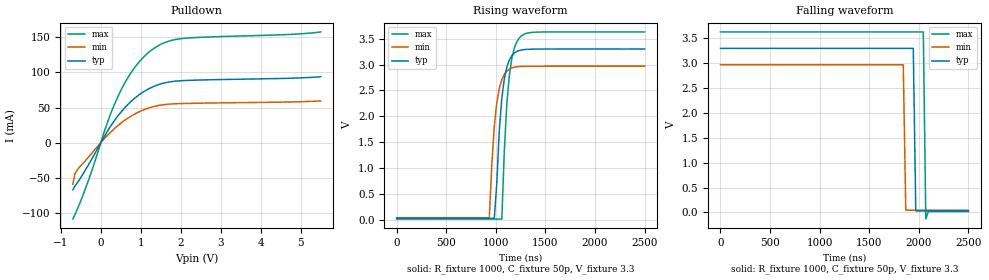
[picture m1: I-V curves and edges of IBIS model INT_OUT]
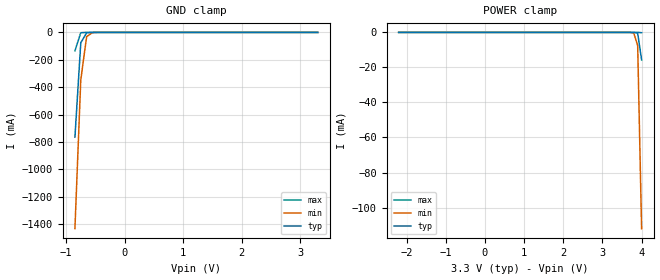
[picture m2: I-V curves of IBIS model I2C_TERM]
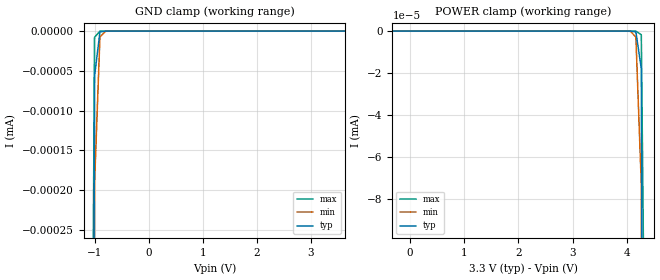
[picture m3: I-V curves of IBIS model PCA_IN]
|   NXP Semiconductors Inc.
|   Specialty Logic Products Group
|   IBIS model of PCA9545B
|   4-Channel I2C switch with
|   interrupt logic and reset
[IBIS Ver]   3.2
[Comment Char]   |_char
|  VDD Typ: 3.3V, Min: 2.97V, Max: 3.63V
[File name]   pca9545b_3_3v.ibs
[File Rev]   1.0
[Date]   Dec 05, 2007 1:30:50 PM
[Source]
Generated by Seshadri Venkataramanan with IbisToolKit at Tempe, AZ
[Notes]
[Disclaimer]
(C) Copyright 2007 NXP Semiconductors
All rights reserved
NXP Semiconductors (NXP) does not warrant that this model and any other
accompanying information (Model) accurately or fully represents the
operating characteristics and specifications of the semiconductor
products to which the Model relates.  Moreover, the Model is furnished
on an "as is" and with "all faults" basis, and without support or
warranty of any kind.  NXP disclaims all warranties, whether expressed
or implied or statutory, including without limitation all implied
warranties of non-infringement, merchantability and fitness for any
purpose, and those arising from a course of dealing or usage of trade.
NXP does not convey any license under its or any third party's patents,
copyrights or other intellectual property or proprietary rights.
You and your company assume any and all risks and liability arising out
of the application or use of the Model.
In no event shall NXP be liable for any direct, indirect, special,
consequential or incidental damages, however caused, whether in
warranty, contract or tort (including negligence), strict liability or
other legal theory, including, without limitation, for lost profits,
business interruption, or corruption or loss of data or information,
arising out of or in connection with the use of or the inability to use
the Model, even if NXP has been advised of the possibility of such
damages.
NXP provides the Model as a courtesy to our customers. You and your
company shall not distribute, convey, sell, or give the Model to anyone
else without receiving prior written permission from NXP.
NXP reserves the right to make changes without notice to the Model to
improve reliability, function, or design.
Please be aware that your receipt and subsequent use of the Model shall
serve as acceptance of these terms and conditions.  If you do not
accept these terms, return or destroy the Model immediately.
[Copyright]
2007
[Component]   PCA9545AD
Si_location Pin
Timing_location Pin
[Manufacturer]   NXP Semiconductors
[Package]
|   variable   typ   min   max
R_pkg   5.95E-02   5.36E-02   6.59E-02
L_pkg   4.21E-09   3.07E-09   5.91E-09
C_pkg   0.910E-12   0.758E-12   1.110E-12
|   SO20
[Pin] signal_name   model_name   R_pin   L_pin   C_pin
1   A0   PCA_IN   5.75E-02  5.91E-09  1.050E-12
2   A1   PCA_IN   6.25E-02  4.85E-09  1.040E-12
3   RESETB   PCA_IN   6.59E-02  3.92E-09  0.861E-12
4   INT0B   INT_IN   5.79E-02  3.32E-09  0.803E-12
5   SD0   I2C_TERM   5.36E-02  3.07E-09  0.758E-12
6   SC0   I2C_TERM   5.36E-02  3.07E-09  0.758E-12
7   INT1B   INT_IN   5.79E-02  3.32E-09  0.803E-12
8   SD1   I2C_TERM   6.59E-02  3.92E-09  0.861E-12
9   SC1   I2C_TERM   6.25E-02  4.85E-09  1.040E-12
10   Vss   GND   5.75E-02  5.91E-09  1.110E-12
11   INT2B   INT_IN   5.75E-02  5.91E-09  1.110E-12
12   SD2   I2C_TERM   6.25E-02  4.85E-09  1.040E-12
13   SC2   I2C_TERM   6.59E-02  3.92E-09  0.861E-12
14   INT3B   INT_IN   5.79E-02  3.32E-09  0.803E-12
15   SD3   I2C_TERM   5.36E-02  3.07E-09  0.758E-12
16   SC3   I2C_TERM   5.36E-02  3.07E-09  0.758E-12
17   INTB   INT_OUT   5.79E-02  3.32E-09  0.803E-12
18   SCL   I2C_TERM   6.59E-02  3.92E-09  0.861E-12
19   SDA   I2C_TERM   6.25E-02  4.85E-09  1.040E-12
20   Vdd   POWER   5.75E-02  5.91E-09  1.110E-12
[Component]   PCA9545APW
Si_location Pin
Timing_location Pin
[Manufacturer]   NXP Semiconductors
[Package]
|   variable   typ   min   max
R_pkg   7.24E-02   6.63E-02   8.34E-02
L_pkg   2.47E-09   2.09E-09   3.18E-09
C_pkg   0.341E-12   0.282E-12   0.420E-12
|   TSSOP20
[Pin] signal_name   model_name   R_pin   L_pin   C_pin
1   A0   PCA_IN   6.63E-02  3.18E-09  0.408E-12
2   A1   PCA_IN   6.67E-02  2.55E-09  0.398E-12
3   RESETB   PCA_IN   8.34E-02  2.35E-09  0.317E-12
4   INT0B   INT_IN   7.44E-02  2.16E-09  0.293E-12
5   SD0   I2C_TERM   7.10E-02  2.09E-09  0.282E-12
6   SC0   I2C_TERM   7.10E-02  2.09E-09  0.282E-12
7   INT1B   INT_IN   7.44E-02  2.16E-09  0.293E-12
8   SD1   I2C_TERM   8.34E-02  2.35E-09  0.317E-12
9   SC1   I2C_TERM   6.67E-02  2.55E-09  0.397E-12
10   Vss   GND   6.63E-02  3.18E-09  0.420E-12
11   INT2B   INT_IN   6.63E-02  3.17E-09  0.420E-12
12   SD2   I2C_TERM   6.67E-02  2.55E-09  0.397E-12
13   SC2   I2C_TERM   8.34E-02  2.35E-09  0.317E-12
14   INT3B   INT_IN   7.44E-02  2.16E-09  0.293E-12
15   SD3   I2C_TERM   7.10E-02  2.09E-09  0.282E-12
16   SC3   I2C_TERM   7.10E-02  2.09E-09  0.282E-12
17   INTB   INT_OUT   7.44E-02  2.16E-09  0.293E-12
18   SCL   I2C_TERM   8.34E-02  2.35E-09  0.317E-12
19   SDA   I2C_TERM   6.67E-02  2.55E-09  0.398E-12
20   Vdd   POWER   6.63E-02  3.17E-09  0.420E-12
[Component]   PCA9545ABS
Si_location Pin
Timing_location Pin
[Manufacturer]   NXP Semiconductors
[Package]
|   variable   typ   min   max
R_pkg   0.364   0.215   0.513
L_pkg   1.49E-09   1.04E-09   1.93E-09
C_pkg   0.149E-12   0.124E-12   0.173E-12
|   HVQFN20
[Package Model]   hvqfn20
[Pin] signal_name   model_name
1   RESETB   I2C_TERM
2   INT0B   INT_IN
3   SD0   I2C_TERM
4   SC0   I2C_TERM
5   INT1B   INT_IN
6   SD1   I2C_TERM
7   SC1   I2C_TERM
8   Vss   GND
9   INT2B   INT_IN
10   SD2   I2C_TERM
11   SC2   I2C_TERM
12   INT3B   INT_IN
13   SD3   I2C_TERM
14   SC3   I2C_TERM
15   INTB   INT_OUT
16   SCL   I2C_TERM
17   SDA   I2C_TERM
18   Vdd   POWER
19   A0   PCA_IN
20   A1   PCA_IN
[Series Pin Mapping] pin_2 model_name   function_table_group
18   6   PCA_SW   1
18   9   PCA_SW   2
18   13   PCA_SW   3
18   16   PCA_SW   4
19   5   PCA_SW   1
19   8   PCA_SW   2
19   12   PCA_SW   3
19   15   PCA_SW   4
[Series Switch Groups]
|   Function Group States
|  default
Off 1 2 3 4 /
On 1 /
On 2 /
On 3 /
On 4 /
[Define Package Model]   hvqfn20
[Manufacturer]   Unknown
[OEM]   Unknown
[Description]   none
[Number of Pins]   20
[Pin Numbers]
|   1 = RESETB
1
|   2 = INT0B
2
|   3 = SD0
3
|   4 = SC0
4
|   5 = INT1B
5
|   6 = SD1
6
|   7 = SC1
7
|   8 = VSS
8
|   9 = INT2B
9
|   10 = SD2
10
|   11 = SC2
11
|   12 = INT3B
12
|   13 = SD3
13
|   14 = SC3
14
|   15 = INTB
15
|   16 = SCL
16
|   17 = SDA
17
|   18 = VDD
18
|   19 = A0
19
|   20 = A1
20
[Model Data]
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[End Model Data]
[End Package Model]
[Model]   PCA_SW
Model_type Series_switch
C_comp   0.5p   0.5p   0.5p
[Temperature Range] 27   -40   85
[Voltage Range]   3.3   2.3   5.5
[Pullup Reference]  3.3   2.3   5.5
[Pulldown Reference]0   0   0
[On]
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[Off]
|   variable   R(typ)   R(min)   R(max)
[R Series]   1e06   1e06   1e06
|[End   PCA_SW
| [End   PCA_SW
| Models and submodels in the file (5): INT_OUT (Open_drain), I2C_TERM (Terminator), PCA_IN (Input), INT_IN (Input), PCA_SW (Series_switch)
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[Model]   INT_OUT
Model_type Open_drain
Vref=3.3
Vmeas=1.65
Rref=1000
Cref=1p
C_comp   2.2p   2p   2.3p
[Model Spec]
Vmeas   1.65   1.485   1.815
[Temperature Range] 27   85   -40
[Voltage Range]   3.3   2.97   3.63
[Pullup Reference]  3.3   2.97   3.63
[Pulldown Reference]0   0   0
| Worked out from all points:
|   slope of the pulldown table from 0 to 0.495 V, typ, clamps not added: 11.6 ohm
|   falling waveform, R_fixture 1000, C_fixture 50p, V_fixture 3.3: 20-80 % time 15.2ns typ, 15.2ns min, 14.5ns max; typ from 3.3 V to 0.031 V
|   rising waveform, R_fixture 1000, C_fixture 50p, V_fixture 3.3: 20-80 % time 71.8ns typ, 71.9ns min, 71ns max; typ from 0.031 V to 3.3 V
[Pulldown]
-700mV    -67.14mA   -59.47mA   -108.7mA
-650mV    -62.1mA    -44.39mA   -102.8mA
-550mV    -53.93mA   -35.7mA    -89.59mA
-250mV    -25.66mA   -16.67mA   -43.97mA
200mV     19.5mA     12.35mA    34.12mA
450mV     39.67mA    25.34mA    68.32mA
600mV     49.71mA    31.88mA    84.94mA
850mV     63.34mA    40.77mA    107.1mA
1.25V     78.11mA    50.21mA    130.9mA
1.6V      85.07mA    54.21mA    142.4mA
2.05V     88.25mA    55.7mA     148.2mA
5.5V      93.73mA    59.3mA     157.5mA
[Falling Waveform]
R_fixture=1000
C_fixture=50p
V_fixture=3.3
V_fixture_min=2.97
V_fixture_max=3.63
0s        3.3V       2.97V      3.63V
1.843us   3.3V       2.97V      3.63V
1.869us   3.3V       53.23mV    3.63V
1.944us   3.3V       45.02mV    3.63V
1.97us    32.62mV    45.02mV    3.63V
2.045us   31.48mV    45.02mV    3.63V
2.071us   31.48mV    45.02mV    -131.3mV
2.096us   31.48mV    45.02mV    19.54mV
2.5us     31.48mV    45.02mV    19.53mV
[Rising Waveform]
R_fixture=1000
C_fixture=50p
V_fixture=3.3
V_fixture_min=2.97
V_fixture_max=3.63
0s        31.48mV    45.02mV    19.55mV
934.3ns   31.49mV    45.09mV    19.56mV
984.8ns   31.5mV     1.815V     19.55mV
1.061us   2.352V     2.712V     20.15mV
1.086us   2.725V     2.814V     1.341V
1.111us   2.952V     2.875V     2.243V
1.136us   3.089V     2.912V     2.79V
1.187us   3.222V     2.949V     3.322V
1.263us   3.283V     2.965V     3.561V
2.5us     3.3V       2.97V      3.63V
[Ramp]
R_load=1000
dV/dt_r   1.961E+0/1.306E-9   1.755E+0/1.384E-9   2.166E+0/1.192E-9
dV/dt_f   1.961E+0/7.920E-10   1.755E+0/1.468E-9   2.166E+0/6.141E-10
|[End   INT_OUT
| [End   I2C_TERM
|  [End   I2C_TERM
[Model]   I2C_TERM
Model_type Terminator
C_comp   9.5p   9.5p   9.5p
[Temperature Range] 27   85   -40
[Voltage Range]   3.3   2.97   3.63
[Pullup Reference]  3.3   2.97   3.63
[Pulldown Reference]0   0   0
[POWER Clamp Reference]3.3   2.97   3.63
[GND Clamp Reference]0   0   0
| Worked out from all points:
|   GND clamp passes 1 mA (typ) near -0.59 V on its own axis
[GND Clamp]
|   -6.000000E-1   -1.554225E-1   -1.242642E-1   -2.666059E-1
|   -5.000000E-1   -1.602113E-1   -1.179351E-1   -2.662641E-1
|   -4.000000E-1   -1.574088E-1   -1.099432E-1   -2.800035E-1
-850mV    -764.8mA   -1.432A    -134.5mA
-750mV    -76.3mA    -346.9mA   -1.957mA
-650mV    -2.644mA   -30.67mA   -13.81uA
-550mV    -57.52uA   -1.64mA    -95.33nA
-450mV    -1.205uA   -66.11uA   -744.9pA
3.3V      580.2pA    638.9pA    606.2pA
[POWER Clamp]
-2.2V     805.5pA    906.8pA    826.1pA
3.8V      -8.329uA   -332.4uA   -8.003nA
3.9V      -395.5uA   -7.559mA   -1.147uA
4V        -15.71mA   -112.1mA   -166.1uA
[Model]   PCA_IN
Model_type Input
Vinh=2.1
Vinl=0.9
C_comp   1.73p   1.73p   1.73p
[Temperature Range] 27   85   -40
[Voltage Range]   3.3   2.97   3.63
[POWER Clamp Reference]3.3   2.97   3.63
[GND Clamp Reference]0   0   0
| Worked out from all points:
|   GND clamp passes 1 mA (typ) near -1.21 V on its own axis
[GND Clamp]
-3.3V     -35.52A    -34.27A    -37.05A
-1.1V     -2.718uA   -4.916uA   -1.14uA
-1V       -56.9nA    -192.5nA   -7.858nA
-900mV    -1.192nA   -7.538nA   -55.05pA
-800mV    -25.74pA   -295.9pA   -1.173pA
-700mV    -1.222pA   -12.26pA   -702.6fA
3.63V     3.63pA     3.63pA     3.63pA
[POWER Clamp]
-330mV    3.63pA     3.63pA     3.63pA
3.97V     -833.7fA   -5.042pA   -670.6fA
4.07V     -8.589pA   -112.4pA   -853.8fA
4.17V     -374.3pA   -2.852nA   -13.03pA
4.27V     -17.84nA   -72.82nA   -1.766nA
4.37V     -852.2nA   -1.86uA    -256.1nA
6.57V     -34.93A    -33.68A    -36.46A
